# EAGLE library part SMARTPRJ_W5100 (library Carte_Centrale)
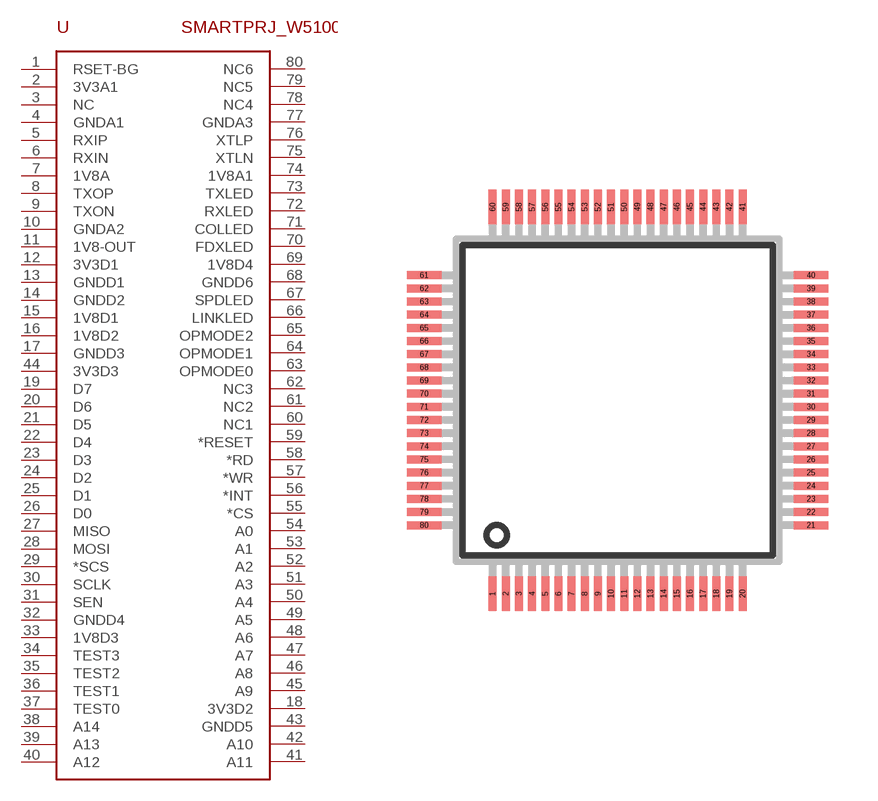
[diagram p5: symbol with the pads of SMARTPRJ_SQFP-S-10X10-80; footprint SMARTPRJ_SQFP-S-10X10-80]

Designator prefix -

## SMARTPRJ_W5100  [SMARTPRJ_SQFP-S-10X10-80]
1  RSET-BG  in
2  3V3A1  pwr
3  NC  nc
4  GNDA1  pwr
5  RXIP  in
6  RXIN  in
7  1V8A  pwr
8  TXOP  out
9  TXON  out
10  GNDA2  pwr
11  1V8-OUT  pwr
12  3V3D1  pwr
13  GNDD1  pwr
14  GNDD2  pwr
15  1V8D1  pwr
16  1V8D2  pwr
17  GNDD3  pwr
18  3V3D2  pwr
19  D7  in
20  D6  in
21  D5  in
22  D4  in
23  D3  in
24  D2  in
25  D1  in
26  D0  in
27  MISO  in
28  MOSI  out
29  *SCS  in
30  SCLK  in
31  SEN  in
32  GNDD4  pwr
33  1V8D3  pwr
34  TEST3  in
35  TEST2  in
36  TEST1  in
37  TEST0  in
38  A14  in
39  A13  in
40  A12  in
41  A11  in
42  A10  in
43  GNDD5  pwr
44  3V3D3  pwr
45  A9  in
46  A8  in
47  A7  in
48  A6  in
49  A5  in
50  A4  in
51  A3  in
52  A2  in
53  A1  in
54  A0  in
55  *CS  in
56  *INT  in
57  *WR  in
58  *RD  in
59  *RESET  in
60  NC1  nc
61  NC2  nc
62  NC3  nc
63  OPMODE0  in
64  OPMODE1  in
65  OPMODE2  in
66  LINKLED  out
67  SPDLED  out
68  GNDD6  pwr
69  1V8D4  pwr
70  FDXLED  out
71  COLLED  out
72  RXLED  out
73  TXLED  out
74  1V8A1  pwr
75  XTLN  out
76  XTLP  out
77  GNDA3  pwr
78  NC4  nc
79  NC5  nc
80  NC6  nc

## Footprint SMARTPRJ_SQFP-S-10X10-80 (pad centres in mm)
QFP80 shrink quad flat pack, square
smd 0.241 x 1.041: 1 -3.8,-5.879; 2 -3.4,-5.879; 3 -3,-5.879; 4 -2.6,-5.879; 5 -2.2,-5.879; 6 -1.8,-5.879; 7 -1.4,-5.879; 8 -1,-5.879; 9 -0.6,-5.879; 10 -0.2,-5.879; 11 0.2,-5.879; 12 0.6,-5.879; 13 1,-5.879; 14 1.4,-5.879; 15 1.8,-5.879; 16 2.2,-5.879; 17 2.6,-5.879; 18 3,-5.879; 19 3.4,-5.879; 20 3.8,-5.879; 41 3.8,5.879; 42 3.4,5.879; 43 3,5.879; 44 2.6,5.879; 45 2.2,5.879; 46 1.8,5.879; 47 1.4,5.879; 48 1,5.879; 49 0.6,5.879; 50 0.2,5.879; 51 -0.2,5.879; 52 -0.6,5.879; 53 -1,5.879; 54 -1.4,5.879; 55 -1.8,5.879; 56 -2.2,5.879; 57 -2.6,5.879; 58 -3,5.879; 59 -3.4,5.879; 60 -3.8,5.879
smd 1.041 x 0.241: 21 5.879,-3.8; 22 5.879,-3.4; 23 5.879,-3; 24 5.879,-2.6; 25 5.879,-2.2; 26 5.879,-1.8; 27 5.879,-1.4; 28 5.879,-1; 29 5.879,-0.6; 30 5.879,-0.2; 31 5.879,0.2; 32 5.879,0.6; 33 5.879,1; 34 5.879,1.4; 35 5.879,1.8; 36 5.879,2.2; 37 5.879,2.6; 38 5.879,3; 39 5.879,3.4; 40 5.879,3.8; 61 -5.879,3.8; 62 -5.879,3.4; 63 -5.879,3; 64 -5.879,2.6; 65 -5.879,2.2; 66 -5.879,1.8; 67 -5.879,1.4; 68 -5.879,1; 69 -5.879,0.6; 70 -5.879,0.2; 71 -5.879,-0.2; 72 -5.879,-0.6; 73 -5.879,-1; 74 -5.879,-1.4; 75 -5.879,-1.8; 76 -5.879,-2.2; 77 -5.879,-2.6; 78 -5.879,-3; 79 -5.879,-3.4; 80 -5.879,-3.8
